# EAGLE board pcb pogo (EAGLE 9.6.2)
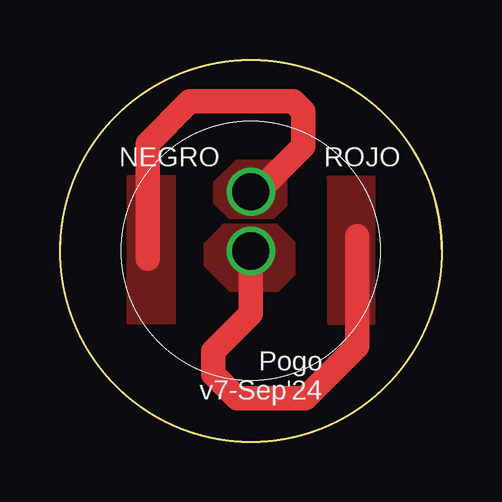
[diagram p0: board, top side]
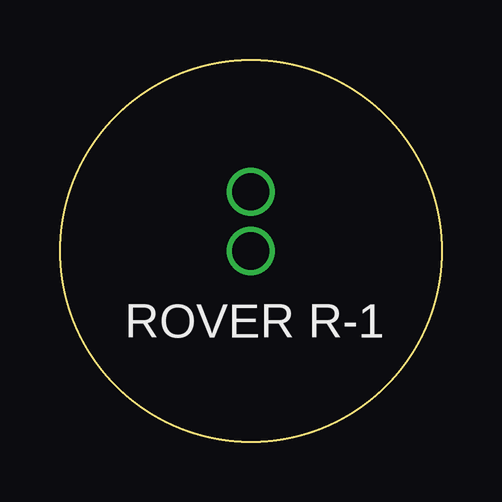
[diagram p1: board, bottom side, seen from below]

Size 15.9 x 15.91 mm. Coordinates in mm from the lower left corner, seen from the top.
Outline: 15.9,7.81 arc182 0,7.81
Outline: circle at 7.95,7.95 radius 7.95
Copper layers (1*16): Top 0.035mm / dielectric 1.5mm / Bottom 0.035mm
Design rules "default *": minimum track width 6mil, minimum drill 0.35mm, track to track 6mil, track to pad 6mil, pad to pad 6mil, via to via 6mil, smd to smd 6mil, copper to edge 1mil, drill to drill 1mil, minimum pad ring 1mil, minimum via ring 1mil, stop-mask expansion 4mil, vias tented up to drill 0mil, thermal gap 10mil

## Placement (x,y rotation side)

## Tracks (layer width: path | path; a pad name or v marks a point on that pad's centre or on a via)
NEG-  (via drill 1.55)
  Top 1.016: 3.65,7.64 3.65,12.43 5.41,14.19 9.71,14.19 10.13,13.77 10.13,12.32 8.13,10.32 8.05,10.32 v7.95,10.42
  pour Top (isolate 0.254): 7.34,11.74 6.39,10.79 6.39,9.96 7.04,9.31 8.91,9.31 9.47,9.87 9.47,11.28 9.01,11.74
  pour Top: 4.75,4.97 2.84,4.97 2.84,11.05 4.75,11.05
POS+  (via drill 1.55)
  Top 1.016: v7.95,7.95 7.95,5.34 6.39,3.78 6.39,2.82 7.39,1.82 10.21,1.82 12.38,3.99 12.38,8.57
  pour Top: 11.16,11.03 13.06,11.03 13.06,4.95 11.19,4.95 11.19,10.93 11.24,10.98
  pour Top: 6.8,9.02 9.01,9.02 9.74,8.29 9.74,6.99 9.06,6.31 7.1,6.31 6.04,7.37 6.04,8.24 6.77,8.97 6.79,8.97

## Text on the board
bPlace: ROVER R-1
tNames: NEGRO | ROJO | Pogo / v7-Sep'24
